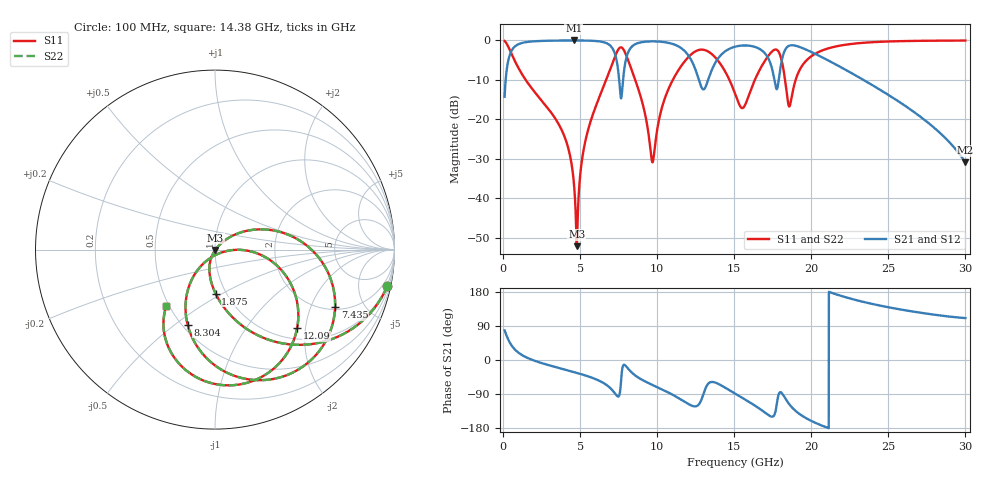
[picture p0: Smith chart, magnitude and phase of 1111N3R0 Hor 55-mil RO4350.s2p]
# GHz S MA R 50
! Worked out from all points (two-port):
!   3201 points, 100 MHz to 30 GHz, reference 50 ohm
!   highest |S21| = -0.02 dB at 4.585 GHz (marker M1); lowest = -30.9 dB at 30 GHz (marker M2)
!   |S21| within 3 dB of the highest: 503.8 MHz to 7.224 GHz (6.721 GHz wide, 174 % of centre); 8.118 GHz to 11.86 GHz (3.745 GHz wide, 37.5 % of centre)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
!   lowest |S11| = -52.1 dB at 4.781 GHz (marker M3), VSWR 1.00, Z = 50.2 - j0.158 ohm
!   |S11| at or under -10 dB: 1.465 GHz to 6.692 GHz (5.226 GHz wide, 128 % of centre); 8.573 GHz to 11.02 GHz (2.444 GHz wide, 25 % of centre); 14.69 GHz to 16.34 GHz (1.653 GHz wide, 10.7 % of centre)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
!   |S22| runs from -52.1 to -0.1 dB; largest |S21 - S12| = 0
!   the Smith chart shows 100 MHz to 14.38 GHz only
!   S11 on the Smith chart (normalised r, x): 100 MHz: 0.89, -9.52; 1.875 GHz: 0.89, -0.47; 7.435 GHz: 2.11, -3.02; 8.304 GHz: 0.53, -0.56; 12.09 GHz: 1.24, -1.80; 14.38 GHz: 0.48, -0.37
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0.1  0.981 -11.9  0.1935 78.1  0.1935 78.1  0.981 -11.9
1.875312  0.2452 -89.2  0.9683 0.6  0.9683 0.6  0.2452 -89.2
3.884219  0.06762 -112.6  0.9957 -23.9  0.9957 -23.9  0.06762 -112.6
4.585  0.0164 -114.0  0.9971 -31.7  0.9971 -31.7  0.0164 -114.0
4.781219  0.002475 -39.5  0.997 -34.0  0.997 -34.0  0.002475 -39.5
5.089563  0.02761 46.0  0.996 -37.7  0.996 -37.7  0.02761 46.0
6.8275  0.3703 15.7  0.8966 -69.4  0.8966 -69.4  0.3703 15.7
7.434844  0.7423 -25.6  0.4648 -96.1  0.4648 -96.1  0.7423 -25.6
7.79925  0.7732 -70.2  0.3352 -13.9  0.3352 -13.9  0.7732 -70.2
8.303812  0.4446 -110.1  0.8123 -31.3  0.8123 -31.3  0.4446 -110.1
9.658656  0.02965 -80.9  0.9704 -65.2  0.9704 -65.2  0.02965 -80.9
10.06978  0.0883 -2.5  0.9659 -72.9  0.9659 -72.9  0.0883 -2.5
12.08803  0.6322 -43.6  0.6179 -117.5  0.6179 -117.5  0.6322 -43.6
13.01306  0.7599 -84.4  0.2392 -88.4  0.2392 -88.4  0.7599 -84.4
14.37725  0.4141 -130.8  0.7179 -72.2  0.7179 -72.2  0.4141 -130.8
15.05  0.2118 -130.3  0.8306 -88.5  0.8306 -88.5  0.2118 -130.3
16.83466  0.4904 -61.5  0.7346 -134.0  0.7346 -134.0  0.4904 -61.5
17.69428  0.7657 -103.3  0.257 -132.3  0.257 -132.3  0.7657 -103.3
18.60063  0.1477 -96.1  0.8598 -118.2  0.8598 -118.2  0.1477 -96.1
20.03956  0.6365 -77.3  0.7068 -161.5  0.7068 -161.5  0.6365 -77.3
25.01978  0.968 -133.4  0.2028 139.1  0.2028 139.1  0.968 -133.4
30  0.9942 -164.5  0.02845 110.5  0.02845 110.5  0.9942 -164.5
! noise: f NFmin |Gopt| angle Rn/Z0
0.1  0.001451  0.8827  3.281  0.002679
3.417  0.009712  0.4785  26.17  0.003028
6.743  0.05772  0.7967  46.6  0.04965
10.06  0.07123  0.7669  67.9  0.04311
13.39  0.5675  0.9583  87.53  1.605
16.7  0.216  0.8727  105.1  0.1364
20.03  0.1674  0.8141  121  0.04714
23.35  0.2259  0.8475  135.2  0.0476
26.67  0.4146  0.9126  150  0.0719
30  1.443  0.9747  165.2  0.2195
